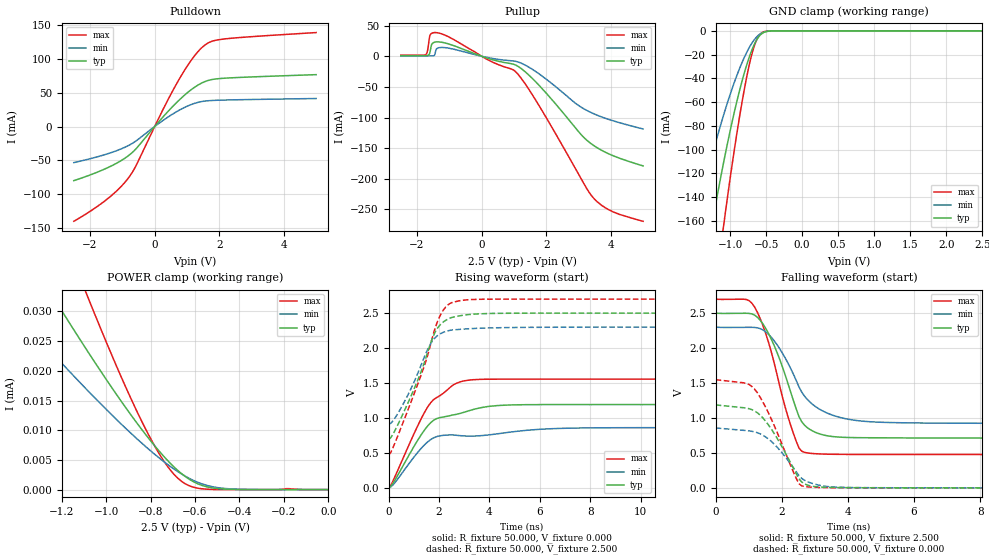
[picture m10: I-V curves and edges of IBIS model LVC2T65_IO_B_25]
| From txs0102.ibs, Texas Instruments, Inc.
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[Model]   LVC2T65_IO_B_25
Model_type  I/O
Vinl=0.15
Vinh=2.3
Enable   Active-High
Vref =   2.5
Rref =   1000000
Cref =   15p
Vmeas =   1.25
| variable   typ   min   max
C_comp   7.13pF   6.12pF   7.81pF
| C_pullup   6.96pF   6.17pF   8.15pF
| C_pulldown   7.90pF   6.77pF   8.89pF
| C_tri-state   7.13pF   6.12pF   7.81pF
[Temperature Range]   40   100   -40
| Ambient temperature   25   85   -40
[Voltage range]   2.5   2.3   2.7
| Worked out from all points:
|   slope of the pulldown table from 0 to 0.375 V, typ, clamps not added: 18.4 ohm
|   slope of the pullup table from 0 to 0.375 V, typ, clamps not added: 59.6 ohm
|   GND clamp passes 1 mA (typ) near -0.52 V on its own axis
|   rising waveform, R_fixture 50.000, V_fixture 0.000: 20-80 % time 1.28ns typ, 1.2ns min, 1.29ns max; typ from 0.003 V to 1.19 V
|   falling waveform, R_fixture 50.000, V_fixture 2.500: 20-80 % time 816ps typ, 1.06ns min, 773ps max; typ from 2.5 V to 0.712 V
|   rising waveform, R_fixture 50.000, V_fixture 2.500: 20-80 % time 1.17ns typ, 1.05ns min, 1.27ns max; typ from 0.697 V to 2.5 V
|   falling waveform, R_fixture 50.000, V_fixture 0.000: 20-80 % time 880ps typ, 898ps min, 860ps max; typ from 1.19 V to 0.003 V
[GND Clamp]
| LVC2T65_IO_B_25
|   Voltage   I(typ)   I(min)   I(max)
-2.5V     -688.5mA   -480.2mA   -942.6mA
-1.49V    -250.3mA   -164.3mA   -364.2mA
-1.25V    -162.9mA   -105.2mA   -240.3mA
-1.1V     -114mA     -72.93mA   -168.7mA
-1.08V    -107.9mA   -68.93mA   -159.6mA
-910mV    -60.46mA   -38.26mA   -87.96mA
-765mV    -27.92mA   -17.63mA   -37.54mA
-655mV    -10.31mA   -6.784mA   -11.18mA
-605mV    -5.221mA   -3.645mA   -4.643mA
-550mV    -1.969mA   -1.526mA   -1.286mA
-350mV    -12.4uA    -18.31uA   -1.425uA
2.5V      292.7pA    2.549nA    59.1pA
[POWER Clamp]
| LVC2T65_IO_B_25
|   Voltage   I(typ)   I(min)   I(max)
-2.5V     115.7uA    78.64uA    183.4uA
-1.48V    47.37uA    32.85uA    71.73uA
-1.25V    33.13uA    23.3uA     48.5uA
-1.095V   23.96uA    17.14uA    33.59uA
-1.07V    22.52uA    16.18uA    31.26uA
-920mV    14.23uA    10.6uA     17.94uA
-805mV    8.461uA    6.695uA    8.956uA
-725mV    4.971uA    4.284uA    3.988uA
-660mV    2.675uA    2.623uA    1.383uA
-585mV    937.8nA    1.195uA    222.4nA
-495mV    158.2nA    316.3nA    13.5nA
0V        0A         0A         0A
[Pulldown]
| LVC2T65_IO_B_25
|   Voltage   I(typ)   I(min)   I(max)
-2.5V     -79.78mA   -53.22mA   -139.7mA
-1.455V   -60.75mA   -40.2mA    -106.5mA
-1.06V    -50.95mA   -33.47mA   -89.59mA
-785mV    -42.06mA   -27.41mA   -74.19mA
-580mV    -33.09mA   -21.41mA   -58.16mA
210mV     11.36mA    7.19mA     20.2mA
710mV     36.64mA    22.63mA    65.45mA
1.14V     54.48mA    32.52mA    98.04mA
1.53V     65.67mA    37.33mA    119.1mA
1.775V    69.21mA    38.35mA    125.6mA
2.215V    71.35mA    39.06mA    129.3mA
5V        76.43mA    41.27mA    138.5mA
[Pullup]
| LVC2T65_IO_B_25
|   Voltage   I(typ)   I(min)   I(max)
-2.5V     987.2uA    519.8uA    1.704mA
-1.735V   1.037mA    505.7uA    2.352mA
-1.675V   1.251mA    505.4uA    8.489mA
-1.595V   7.015mA    509.8uA    34.19mA
-1.535V   20.04mA    533.6uA    37.52mA
-1.455V   22.81mA    1.926mA    38.53mA
-1.39V    23.34mA    12.16mA    38.41mA
985mV     -13.02mA   -7.798mA   -22.48mA
1.68V     -42.03mA   -25.15mA   -72.08mA
3.445V    -144.7mA   -93.22mA   -230.2mA
4.08V     -162.5mA   -105.5mA   -254.1mA
5V        -178.9mA   -118.7mA   -269.3mA
[Ramp]
| LVC2T65_IO_B_25
| variable   typ   min   max
dV/dt_r   0.76/1.29E-09   0.56/1.21E-09   0.99/1.30E-09
dV/dt_f   1.07/8.16E-10   0.82/1.06E-09   1.33/7.74E-10
R_load = 50
[Rising Waveform]
R_fixture = 50.000
V_fixture = 0.000
V_fixture_min = 0.000
V_fixture_max = 0.000
C_fixture = 0.000
L_fixture = 0.000
|  time   V(typ)   V(min)   V(max)
0s        3.332mV    3.083mV    3.488mV
168ps     66.56mV    44.37mV    99.6mV
1.26ns    744.6mV    555.3mV    969.2mV
1.68ns    938.3mV    695.9mV    1.225V
2.1ns     1.012V     750.4mV    1.337V
2.688ns   1.054V     754.3mV    1.497V
3.948ns   1.166V     758.9mV    1.556V
6.384ns   1.193V     846.9mV    1.557V
10.5ns    1.193V     863.2mV    1.557V
419.9ns   1.189V     859.8mV    1.548V
[Falling Waveform]
R_fixture = 50.000
V_fixture = 2.500
V_fixture_min = 2.300
V_fixture_max = 2.700
C_fixture = 0.000
L_fixture = 0.000
|  time   V(typ)   V(min)   V(max)
0s        2.5V       2.3V       2.7V
924ps     2.498V     2.297V     2.695V
1.176ns   2.472V     2.295V     2.588V
1.764ns   2.043V     2.108V     1.799V
2.1ns     1.62V      1.862V     1.16V
2.52ns    1.021V     1.446V     571.5mV
2.94ns    813.5mV    1.193V     493.3mV
3.696ns   729.5mV    1.018V     481.8mV
9.996ns   714.2mV    924.9mV    479.3mV
419.9ns   712.1mV    912.2mV    478.6mV
[Rising Waveform]
R_fixture = 50.000
V_fixture = 2.500
V_fixture_min = 2.300
V_fixture_max = 2.700
C_fixture = 0.000
L_fixture = 0.000
|  time   V(typ)   V(min)   V(max)
0s        697.4mV    912mV      470.9mV
336ps     885mV      1.05V      723mV
924ps     1.346V     1.45V      1.266V
1.428ns   1.807V     1.884V     1.762V
1.68ns    2.087V     2.072V     2.075V
1.848ns   2.232V     2.151V     2.291V
2.1ns     2.353V     2.215V     2.504V
2.52ns    2.439V     2.26V      2.652V
3.78ns    2.492V     2.286V     2.699V
419.9ns   2.5V       2.3V       2.7V
[Falling Waveform]
R_fixture = 50.000
V_fixture = 0.000
V_fixture_min = 0.000
V_fixture_max = 0.000
C_fixture = 0.000
L_fixture = 0.000
|  time   V(typ)   V(min)   V(max)
0s        1.188V     859.1mV    1.548V
924ps     1.142V     821.1mV    1.496V
1.176ns   1.102V     802.6mV    1.414V
1.428ns   1.002V     755mV      1.229V
1.68ns    845.3mV    667.5mV    988.8mV
2.016ns   581.1mV    498.4mV    614.8mV
2.52ns    131.3mV    177.3mV    60.98mV
2.856ns   31.38mV    76.53mV    13.95mV
3.528ns   8.467mV    15.64mV    5.203mV
419.9ns   3.079mV    2.64mV     3.383mV
